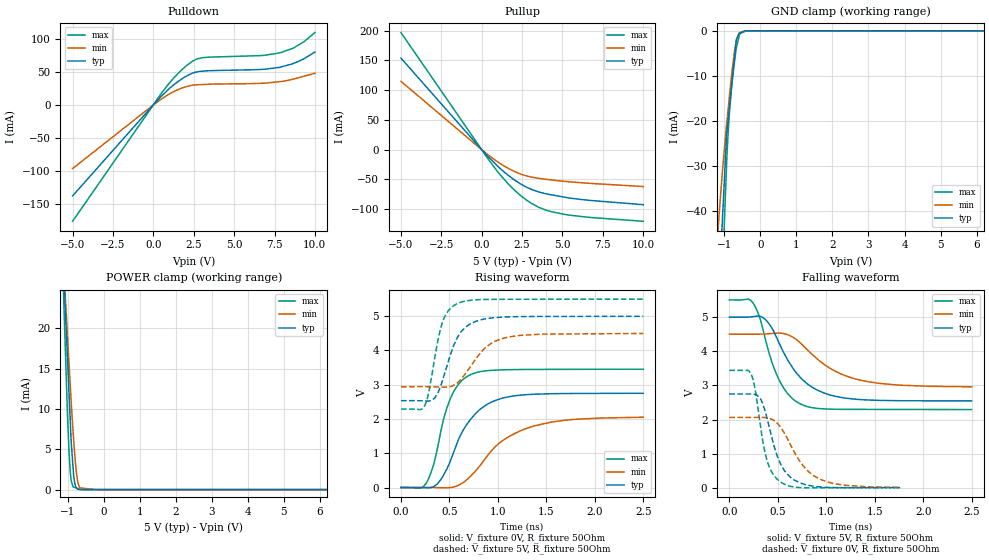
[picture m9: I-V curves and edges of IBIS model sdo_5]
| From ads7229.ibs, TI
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|   sdo_5 Model
[Model]   sdo_5
Model_type   3-state
Polarity   Non-Inverting
Vmeas = 2.5
Vref = 2.5
Cref = 30pF
Rref = 50
|   typ   min   max
|   (nom PVT)   (Fast PVT)   (slow PVT)
|C_comp from frequency sweep method(F=50MHz)
C_comp   4.855e-12   3.896e-12   5.693e-12
|OFF state: BUFFER IN HIGH IMPEDANCE
|C_comp   4.855e-12   3.896e-12   5.693e-12
|ON state : BUFFER OUTPUT TURNED HIGH
|C_comp   5.192e-12   4.233e-12   6.095e-12
|C_comp from LC tank measurement(L=1nH)
|ON state : BUFFER OUTPUT TURNED HIGH
|Resonant Frequency(Hz)   2.480e+09   2.680e+09   2.370e+09
|C_comp   4.123e-12   3.530e-12   4.514e-12
|OFF state: BUFFER IN HIGH IMPEDANCE
|Resonant Frequency   2.600e+09   2.850e+09   2.440e+09
|C_comp   3.751e-12   3.122e-12   4.259e-12
| Where nom  PVT is Nominal Process,  5V,  28C
|   Fast PVT is Strong Process,   5.5V,  -40C
|   Slow PVT is Weak Process,   4.5V,  88C
[Voltage Range]   5   4.5   5.5
|Ambient Temperature   25   85   -40
|Junction Temperature
[Temperature Range]   28   88   -40
[Pullup Reference]   5   4.5   5.5
[Pulldown Reference]   0   0   0
[Power Clamp Reference]   5   4.5   5.5
[GND Clamp Reference]   0   0   0
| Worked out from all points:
|   slope of the pulldown table from 0 to 0.75 V, typ, clamps not added: 38.9 ohm
|   slope of the pullup table from 0 to 0.75 V, typ, clamps not added: 35.2 ohm
|   GND clamp passes 1 mA (typ) near -0.62 V on its own axis
|   POWER clamp passes 1 mA (typ) near -0.81 V on its own axis
|   falling waveform, V_fixture 5V, R_fixture 50Ohm: 20-80 % time 339ps typ, 463ps min, 231ps max; typ from 5 V to 2.55 V
|   rising waveform, V_fixture 0V, R_fixture 50Ohm: 20-80 % time 311ps typ, 476ps min, 199ps max; typ from 0 V to 2.75 V
|   rising waveform, V_fixture 5V, R_fixture 50Ohm: 20-80 % time 194ps typ, 273ps min, 135ps max; typ from 2.53 V to 5 V
|   falling waveform, V_fixture 0V, R_fixture 50Ohm: 20-80 % time 184ps typ, 282ps min, 128ps max; typ from 2.75 V to 0.01 V
[Pulldown]
|   Voltage   I(typ)   I(min)   I(max)
-5V       -138.4mA   -96.83mA   -177mA
528mV     14.11mA    9.495mA    18.76mA
1.216V    29.73mA    19.67mA    39.74mA
2.007V    43.3mA     27.58mA    58.86mA
2.38V     47.96mA    29.92mA    65.81mA
2.684V    50.17mA    30.7mA     69.91mA
3.08V     51.49mA    31.09mA    71.99mA
6.6V      53.94mA    32.88mA    75.06mA
7.854V    57.55mA    35.54mA    79.3mA
8.684V    63.33mA    39.47mA    86.72mA
9.35V     70.62mA    43.89mA    96.59mA
10V       80.52mA    48.22mA    110.1mA
[GND Clamp]
|   Voltage   I(typ)   I(min)   I(max)
-5V       -892.6mA   -646.6mA   -1.244A
-1.216V   -69.01mA   -48.87mA   -99.62mA
-1.143V   -55.86mA   -40.33mA   -79.34mA
-1.089V   -47.18mA   -34.62mA   -64.72mA
-1.044V   -40mA      -30.13mA   -53.41mA
-1.001V   -33.15mA   -26.25mA   -42.6mA
-935mV    -22.86mA   -20.46mA   -28.8mA
-863.5mV  -17.25mA   -14.75mA   -18.41mA
-786.5mV  -11.21mA   -8.852mA   -11.26mA
-670mV    -2.069mA   -2.242mA   -3.888mA
-580.5mV  -549.3uA   -384.9uA   -836.4uA
10V       0A         0A         0A
[Pullup]
|   Voltage   I(typ)   I(min)   I(max)
-5V       153.8mA    114.8mA    196.7mA
445.5mV   -13.17mA   -9.806mA   -17.57mA
1.04V     -28.95mA   -21.46mA   -38.79mA
1.672V    -43.61mA   -31.8mA    -58.38mA
2.475V    -58.65mA   -41.69mA   -78.57mA
3.08V     -66.79mA   -46.16mA   -90.21mA
3.52V     -70.95mA   -48.04mA   -96.68mA
4.301V    -75.82mA   -50.92mA   -104.2mA
5.192V    -80.1mA    -53.4mA    -109.1mA
6.6V      -84.95mA   -56.4mA    -113.6mA
10V       -92.49mA   -61.96mA   -120.4mA
[POWER Clamp]
|   Voltage   I(typ)   I(min)   I(max)
-5V       207.8mA    188.7mA    235.2mA
-1.14V    29.98mA    30.25mA    28.15mA
-1.111V   27.05mA    27.69mA    23.81mA
-1.098V   25.73mA    26.55mA    22.03mA
-1.001V   15.92mA    18.78mA    8.86mA
-929.5mV  8.681mA    13.06mA    2.319mA
-900mV    5.812mA    10.7mA     1.118mA
-835mV    1.822mA    6.276mA    318.4uA
-720mV    59.67uA    941.3uA    122.5uA
-666mV    12.26uA    216.5uA    30.46uA
-202.5mV  0A         0A         466.9nA
10V       0A         0A         0A
[Ramp]
R_load = 50
|   typ   min   max
dV/dt_r   1.64965/3.09996e-10   1.23039/4.75166e-10   2.07051/1.98387e-10
dV/dt_f   1.47187/3.38643e-10   0.924529/4.60559e-10   1.92331/2.30886e-10
[Falling Waveform]
V_fixture = 5V
V_fixture_min = 4.5V
V_fixture_max = 5.5V
R_fixture = 50Ohm
|   Time   V(typ)   V(min)   V(max)
0s        5V         4.5V       5.5V
243ps     5.011V     4.499V     5.418V
306ps     5.025V     4.5V       5.049V
372ps     4.928V     4.506V     4.35V
508ps     4.275V     4.532V     3.193V
616ps     3.679V     4.468V     2.714V
745ps     3.197V     4.211V     2.442V
1.038ns   2.723V     3.503V     2.306V
1.367ns   2.583V     3.144V     2.299V
2.5ns     2.547V     2.959V     2.294V
[Rising Waveform]
V_fixture = 0V
V_fixture_min = 0V
V_fixture_max = 0V
R_fixture = 50Ohm
|   Time   V(typ)   V(min)   V(max)
0s        1.65nV     1.848nV    1.527nV
261ps     -6.179mV   636.7uV    125.3mV
373ps     101.3mV    -1.316mV   1.094V
439ps     358.2mV    -5.786mV   1.985V
503ps     726.4mV    -2.083mV   2.545V
593ps     1.394V     64.6mV     3.012V
708ps     1.951V     300.2mV    3.279V
925ps     2.48V      1.043V     3.417V
1.278ns   2.706V     1.706V     3.444V
2.5ns     2.749V     2.051V     3.451V
[Rising Waveform]
V_fixture = 5V
V_fixture_min = 4.5V
V_fixture_max = 5.5V
R_fixture = 50Ohm
|   Time   V(typ)   V(min)   V(max)
0s        2.534V     2.941V     2.288V
247ps     2.525V     2.942V     2.395V
287ps     2.521V     2.941V     2.778V
345ps     2.605V     2.938V     3.724V
424ps     3.078V     2.93V      4.785V
585ps     4.389V     3.058V     5.373V
692ps     4.732V     3.428V     5.454V
872ps     4.922V     4.08V      5.486V
1.093ns   4.978V     4.381V     5.492V
2.5ns     4.995V     4.495V     5.497V
[Falling Waveform]
V_fixture = 0V
V_fixture_min = 0V
V_fixture_max = 0V
R_fixture = 50Ohm
|   Time   V(typ)   V(min)   V(max)
0s        2.748V     2.065V     3.44V
224ps     2.749V     2.066V     3.34V
268ps     2.732V     2.067V     2.853V
324ps     2.594V     2.067V     1.768V
387ps     2.066V     2.054V     826.8mV
443ps     1.424V     2.006V     437.7mV
527ps     711.7mV    1.786V     179.2mV
742ps     137mV      720.8mV    8.974mV
949ps     27.97mV    240.1mV    5.531mV
1.763ns   10.04mV    16.49mV    8.303mV
